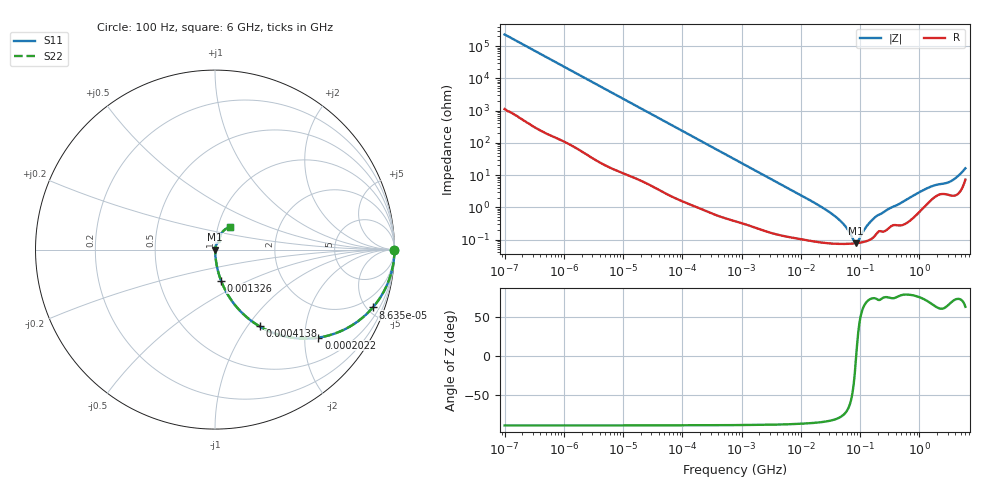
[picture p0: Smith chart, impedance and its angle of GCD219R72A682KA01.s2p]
!Murata Part Number: GCD219R72A682KA01
!These Parameters are Measured in Series Mode Connection
!Data Generated on Mar 13, 2026
!  o--ll--o
!Port1  Port2
!  o------o
!Operation Temp=25[degC], DC Bias Voltage=0[V]
!Freq. Start=100[Hz] Stop=6[GHz] 401[Steps]
# Hz S RI R 50
!Freq.(Hz) S11(Real) S11(Imag) S21(Real) S21(Imag) S12(Real) S12(Imag) S22(Real) S22(Imag)
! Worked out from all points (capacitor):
!   401 points, 100 Hz to 6 GHz, reference 50 ohm
!   read as one part in series: C = 6.9 nF near 109 Hz
!   lowest |Z| = 77 mohm at 85.28 MHz (marker M1)
!   series resonance near 86.06 MHz, so ESL is about 500 pH
!   S11 on the Smith chart (normalised r, x): 100 Hz: open; 86.35 kHz: 1.03, -5.45; 202.2 kHz: 1.02, -2.33; 413.8 kHz: 1.01, -1.14; 1.326 MHz: 1.01, -0.36; 6 GHz: 1.15, +0.29
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100  1 -0.000434  2.3e-06 0.000434  2.3e-06 0.000434  1 -0.000434
2008  0.9999 -0.00864  0.000115 0.00864  0.000115 0.00864  0.9999 -0.00864
12592  0.9968 -0.0538  0.00318 0.0538  0.00318 0.0538  0.9968 -0.0538
40335  0.9703 -0.1667  0.0297 0.1667  0.0297 0.1667  0.9703 -0.1667
86348  0.8796 -0.3223  0.1204 0.3223  0.1204 0.3223  0.8796 -0.3223
202169  0.576 -0.4904  0.424 0.4904  0.424 0.4904  0.576 -0.4904
413847  0.2484 -0.4274  0.7516 0.4274  0.7516 0.4274  0.2484 -0.4274
774597  0.0886 -0.2782  0.9114 0.2782  0.9114 0.2782  0.0886 -0.2782
1325623  0.0338 -0.1732  0.9662 0.1732  0.9662 0.1732  0.0338 -0.1732
3712478  0.00561 -0.0641  0.9944 0.0641  0.9944 0.0641  0.00561 -0.0641
1.555665e7  0.00112 -0.0151  0.9989 0.0151  0.9989 0.0151  0.00112 -0.0151
4.556224e7  0.000748 -0.00388  0.9993 0.00388  0.9993 0.00388  0.000748 -0.00388
5.699437e7  0.000739 -0.00243  0.9993 0.00243  0.9993 0.00243  0.000739 -0.00243
7.797396e7  0.000755 -0.000567  0.9992 0.000567  0.9992 0.000567  0.000755 -0.000567
8.527865e7  0.000767 -5.15e-05  0.9992 5.15e-05  0.9992 5.15e-05  0.000767 -5.15e-05
9.326766e7  0.000783 0.000465  0.9992 -0.000465  0.9992 -0.000465  0.000783 0.000465
1.220122e8  0.000871 0.00207  0.9991 -0.00207  0.9991 -0.00207  0.000871 0.00207
1.596157e8  0.0011 0.00388  0.9989 -0.00388  0.9989 -0.00388  0.0011 0.00388
3.124326e8  0.00241 0.00888  0.9976 -0.00888  0.9976 -0.00888  0.00241 0.00888
1.369159e9  0.014 0.0362  0.986 -0.0362  0.986 -0.0362  0.014 0.0362
3.352442e9  0.0261 0.0561  0.9739 -0.0561  0.9739 -0.0561  0.0261 0.0561
6e9  0.0845 0.1242  0.9155 -0.1242  0.9155 -0.1242  0.0845 0.1242
